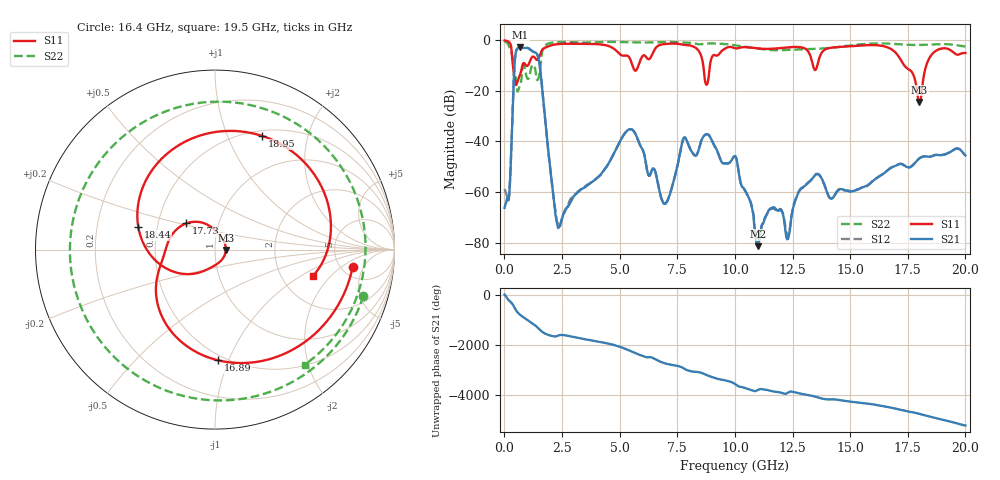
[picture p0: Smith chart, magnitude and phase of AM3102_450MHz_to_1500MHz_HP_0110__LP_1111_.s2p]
!Agilent Technologies,E8364B,MY43040894,A.07.50.67
!Agilent E8364B: A.07.50.67
!Date: Thursday, January 11, 2018 05:50:16
!Correction: S11(Full 2 Port(1,2))
!S21(Full 2 Port(1,2))
!S12(Full 2 Port(1,2))
!S22(Full 2 Port(1,2))
!S2P File: Measurements: S11, S21, S12, S22:
# Hz S  dB  R 50
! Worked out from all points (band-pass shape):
!   1601 points, 10 MHz to 20 GHz, reference 50 ohm
!   highest |S21| = -2.84 dB at 684.7 MHz (marker M1); lowest = -81.4 dB at 11 GHz (marker M2)
!   |S21| within 3 dB of the highest: 478.4 MHz to 1.435 GHz (956.8 MHz wide, 100 % of centre)
!   lowest |S11| = -24.4 dB at 18 GHz (marker M3), VSWR 1.13, Z = 56.4 - j0.294 ohm
!   |S11| at or under -10 dB: 372.1 MHz to 779.5 MHz (407.3 MHz wide, 70.7 % of centre); 8.629 GHz to 8.914 GHz (284.2 MHz wide, 3.24 % of centre); 17.35 GHz to 18.3 GHz (947.7 MHz wide, 5.32 % of centre)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
!   |S22| runs from -20.3 to -0.5 dB; largest |S21 - S12| = 0.0028
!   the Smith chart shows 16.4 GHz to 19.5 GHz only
!   S11 on the Smith chart (normalised r, x): 16.4 GHz: 6.29, -3.06; 16.89 GHz: 0.46, -0.92; 17.73 GHz: 0.70, +0.21; 18.44 GHz: 0.39, +0.12; 18.95 GHz: 0.56, +1.34; 19.5 GHz: 3.00, -1.29
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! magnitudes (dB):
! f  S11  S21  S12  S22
! 10 MHz  -0.1  -66.3  -58.8  -0.5
! 197.4 MHz  -0.7  -62.3  -62.0  -2.3
! 459.8 MHz  -16.0  -7.4  -7.4  -13.3
! 684.7 MHz  -13.5  -2.8  -2.8  -17.7
! 1.484 GHz  -7.1  -7.4  -7.5  -14.8
! 2.309 GHz  -1.5  -73.3  -72.2  -0.7
! 3.346 GHz  -1.4  -58.9  -58.7  -0.9
! 5.457 GHz  -7.4  -35.1  -35.1  -0.8
! 6.682 GHz  -2.1  -57.5  -57.3  -0.7
! 7.819 GHz  -1.8  -38.4  -38.4  -0.9
! 10.01 GHz  -3.1  -45.8  -45.8  -2.0
! 11 GHz  -3.2  -81.4  -81.1  -3.3
! 13.34 GHz  -8.2  -54.9  -54.9  -3.4
! 16.4 GHz  -2.2  -53.0  -52.9  -1.2
! 16.68 GHz  -3.0  -51.0  -50.9  -1.3
! 16.89 GHz  -4.2  -49.9  -49.9  -1.4
! 17.73 GHz  -13.3  -49.3  -49.3  -1.8
! 18 GHz  -24.4  -46.7  -46.7  -1.8
! 18.44 GHz  -7.0  -46.1  -46.0  -1.7
! 18.95 GHz  -3.3  -45.4  -45.4  -1.5
! 19.5 GHz  -4.9  -43.2  -43.3  -1.8
! 20 GHz  -5.0  -45.5  -45.5  -2.5
